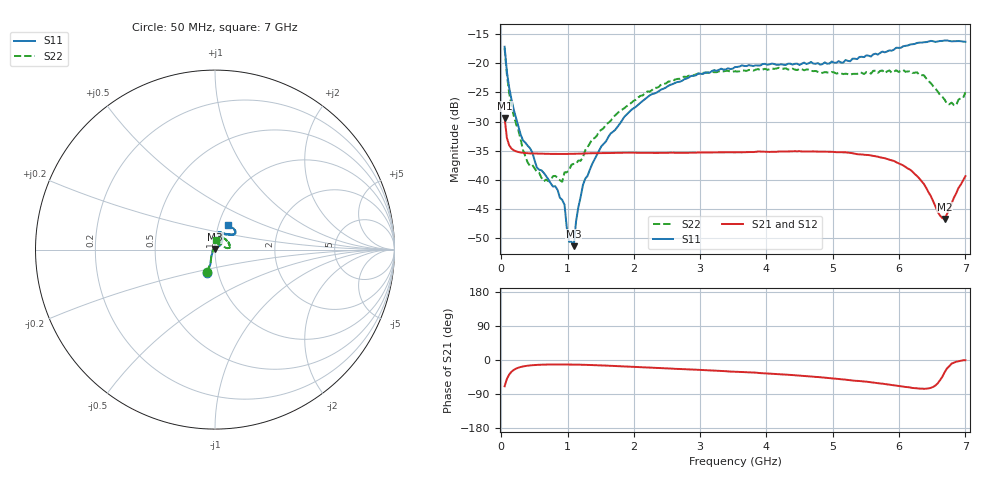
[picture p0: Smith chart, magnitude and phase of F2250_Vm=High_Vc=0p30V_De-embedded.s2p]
! Integrated Device Technology
! Corporate Headquarters
! 6024 Silver Creek Valley Road
! San Jose, CA 95138  USA
! Phone:  1-408-284-8200
! Toll Free:  1-800-223-1366
! Webpage:  http://www.idt.com/
! Timing and RF Division
! 515 Groton Road, Suite 102
! Westford, MA 01886-6024
! Device:  F2250
! Description: Voltage Variable RF Attenuator
! Frequency:  50.0 -  6000.00 MHz
! Package:  3x3 mm Thin QFN Plastic Package: 16 pin
! Ports:  2 RF, 3 DC
!  Pin  1  = GND
!  Pin  2  = NC
!  Pin  3  = RF1  = Port 1
!  Pin  4  = NC
!  Pin  5  = GND
!  Pin  6  = GND
!  Pin  7  = GND
!  Pin  8  = GND
!  Pin  9  = NC
!  Pin 10  = RF2  = Port 2
!  Pin 11  = NC
!  Pin 12  = GND
!  Pin 13  = GND
!  Pin 14  = VCNTRL
!  Pin 15  = VDD
!  Pin 16  = VMODE
! Vcntrl:  0.300 Volts
! Vmode:  +3.300 Volts
! Vdd:  +3.30  Volts
! Current:  1.251 mA
! Data:  The device was measured on a the F2250 evaluation board which has
!  individual transmission lines to the RF pins.  Data was collected
!  using a calibrated network analyzer.  The evaluation board was
!  de-embedded using a TRL calibration technique.
!  The reference plane is the edge of the package pin.
! Misc:  SN 10
!  Action Tracker AT0258
! Date Measured:  2014-11-26
! Date:  2015-10-15  MJV
! Note:
!  Integrated Device Technology supplies this data as a sample of measured
!  data at the package pin for this product.  Your particular data for this
!  product may vary.
!  Data was taken at 25 degrees C.
!  Integrated Device Technology reserves the right to change this data at anytime.
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# GHz S dB R 50
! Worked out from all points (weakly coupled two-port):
!   201 points, 50 MHz to 7 GHz, reference 50 ohm
!   highest |S21| = -29.36 dB at 50 MHz (marker M1); lowest = -46.7 dB at 6.687 GHz (marker M2)
!   lowest |S11| = -51.3 dB at 1.093 GHz (marker M3), VSWR 1.01, Z = 50 + j0.271 ohm
!   |S11| at or under -10 dB: start of sweep to end of sweep
!   |S22| runs from -40.3 to -17.4 dB; largest |S21 - S12| = 6e-05
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0.05  -17.18 -108.5  -29.36 -69.3  -29.36 -69.3  -17.45 -110.2
0.08475  -21.47 -107.4  -32.82 -49.9  -32.82 -49.9  -21.98 -108.1
0.189  -28.00 -120.0  -34.92 -26.1  -34.92 -26.0  -29.06 -122.3
0.29325  -32.26 -127.4  -35.29 -18.4  -35.29 -18.4  -33.11 -130.5
0.3975  -34.12 -142.2  -35.42 -15.0  -35.42 -15.0  -36.98 -155.6
0.5365  -37.87 -154.6  -35.50 -12.9  -35.49 -12.9  -38.65 -178.9
0.64075  -38.78 -162.6  -35.52 -12.2  -35.52 -12.2  -40.22 158.8
0.91875  -43.41 156.1  -35.54 -11.8  -35.54 -11.8  -40.31 121.7
0.9535  -44.23 170.9  -35.54 -11.8  -35.54 -11.8  -38.68 118.9
1.023  -50.60 140.4  -35.53 -11.9  -35.53 -12.0  -38.31 101.5
1.0925  -51.34 89.6  -35.52 -12.0  -35.52 -12.1  -37.25 92.3
1.12725  -47.12 61.7  -35.51 -12.2  -35.50 -12.2  -37.21 85.2
1.2315  -40.85 40.9  -35.47 -12.5  -35.47 -12.5  -36.13 71.2
1.6485  -32.04 41.2  -35.38 -15.3  -35.38 -15.3  -29.89 57.0
2.37825  -24.76 46.7  -35.35 -21.1  -35.35 -21.2  -24.05 52.4
3.525  -20.66 71.7  -35.27 -30.8  -35.27 -30.8  -21.38 72.2
4.7065  -20.06 72.0  -35.11 -44.1  -35.11 -44.1  -21.36 69.9
5.85325  -17.79 40.5  -36.53 -65.0  -36.53 -65.1  -21.23 22.6
6.3745  -16.40 41.0  -40.69 -75.9  -40.71 -76.0  -22.06 6.5
6.68725  -16.11 47.9  -46.67 -32.2  -46.68 -31.8  -26.23 27.8
6.861  -16.22 54.5  -42.29 -4.6  -42.26 -4.6  -27.20 57.5
7  -16.32 62.4  -39.35 -0.7  -39.32 -1.0  -24.97 84.2
